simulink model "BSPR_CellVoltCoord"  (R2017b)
settings: Solver=FixedStepDiscrete  StartTime=0.0  StopTime=10.0  FixedStep=0.02  RelTol=1e-3  EnableMultiTasking=on
undefined symbols (not defined in the file): bin2dec, BSPR_CellVoltVldChkDisbl_C, BSPR_cntCellInvldNum_C, BSPR_cntCellSerNum_C, BSPR_cntCellVoltOutRngDiag_CW, BSPR_cntCellVoltVldDiag_CW, BSPR_cntCellVoltVldHi_C, BSPR_cntVoltCellAvl_C, BSPR_iCellVoltDeltaBattCurr_X, BSPR_rCellVoltDeltaBattSOC_Y, BSPR_tBattTempForCellHi_C, BSPR_tBattTempForCellLo_C, BSPR_tiCellVoltInvldChk_C, BSPR_tiCellVoltInvldChkdT_C, BSPR_tiCellVoltRngHiChk_C, BSPR_tiCellVoltRngHiChkdT_C, BSPR_tiCellVoltRngLoChk_C, BSPR_tiCellVoltRngLoChkdT_C, BSPR_uCellVoltDelta_Z, BSPR_uCellVoltHi_C, BSPR_uCellVoltLo_C, BSPR_uCellVoltMaxLim_C, BSPR_uCellVoltMinLim_C
libraries: simulink x35, AIWAYS_Powertrain_BMS_lib x2
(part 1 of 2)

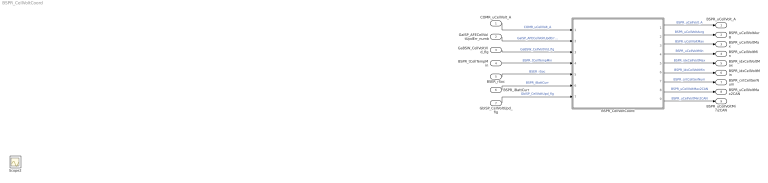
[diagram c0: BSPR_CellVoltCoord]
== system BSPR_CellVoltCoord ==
  COMR_uCellVolt_A : Inport
  GaISP_AFECellVoltUpdErr_numb : Inport  Port=2
  GaBSW_CellVoltVld_flg : Inport  Port=3
  BSPR_tCellTempMin : Inport  Port=4
  BSER_rSoc : Inport  Port=5
  BSPR_iBattCurr : Inport  Port=6
  GbISP_CellVoltUpd_flg : Inport  Port=7
  BSPR_CellVoltCoord : Subsystem
  BSPR_uCellVolt_A : Outport
  BSPR_uCellVoltAvrg : Outport  Port=2
  BSPR_uCellVoltMax : Outport  Port=3
  BSPR_uCellVoltMin : Outport  Port=4
  BSPR_idxCellVoltMax : Outport  Port=5
  BSPR_idxCellVoltMin : Outport  Port=6
  BSPR_cntCellSerNum : Outport  Port=7
  BSPR_uCellVoltMax2CAN : Outport  Port=8
  BSPR_uCellVoltMin2CAN : Outport  Port=9
  Scope2 : Scope
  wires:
  COMR_uCellVolt_A/1 -> BSPR_CellVoltCoord/1(COMR_uCellVolt_A)  "COMR_uCellVolt_A"
  BSPR_CellVoltCoord/1(BSPR_uCellVolt_A) -> BSPR_uCellVolt_A/1  "BSPR_uCellVolt_A"
  BSPR_CellVoltCoord/2(BSPR_uCellVoltAvrg) -> BSPR_uCellVoltAvrg/1  "BSPR_uCellVoltAvrg"
  BSPR_CellVoltCoord/3(BSPR_uCellVoltMax) -> BSPR_uCellVoltMax/1  "BSPR_uCellVoltMax"
  BSPR_CellVoltCoord/4(BSPR_uCellVoltMin) -> BSPR_uCellVoltMin/1  "BSPR_uCellVoltMin"
  BSPR_CellVoltCoord/5(BSPR_idxCellVoltMax) -> BSPR_idxCellVoltMax/1  "BSPR_idxCellVoltMax"
  BSPR_CellVoltCoord/6(BSPR_idxCellVoltMin) -> BSPR_idxCellVoltMin/1  "BSPR_idxCellVoltMin"
  GaISP_AFECellVoltUpdErr_numb/1 -> BSPR_CellVoltCoord/2(GaISP_AFECellVoltUpdErr_numb)  "GaISP_AFECellVoltUpdErr_numb"
  BSPR_CellVoltCoord/7(BSPR_cntCellSerNum) -> BSPR_cntCellSerNum/1  "BSPR_cntCellSerNum"
  GaBSW_CellVoltVld_flg/1 -> BSPR_CellVoltCoord/3(GaBSW_CellVoltVld_flg)  "GaBSW_CellVoltVld_flg"
  BSPR_tCellTempMin/1 -> BSPR_CellVoltCoord/4(BSPR_tCellTempMin)  "BSPR_tCellTempMin"
  BSER_rSoc/1 -> BSPR_CellVoltCoord/5(BSER_rSoc)  "BSER_rSoc"
  BSPR_iBattCurr/1 -> BSPR_CellVoltCoord/6(BSPR_iBattCurr)  "BSPR_iBattCurr"
  BSPR_CellVoltCoord/8(BSPR_uCellVoltMax2CAN) -> BSPR_uCellVoltMax2CAN/1  "BSPR_uCellVoltMax2CAN"
  BSPR_CellVoltCoord/9(BSPR_uCellVoltMin2CAN) -> BSPR_uCellVoltMin2CAN/1  "BSPR_uCellVoltMin2CAN"
  GbISP_CellVoltUpd_flg/1 -> BSPR_CellVoltCoord/7(GbISP_CellVoltUpd_flg)  "GbISP_CellVoltUpd_flg"

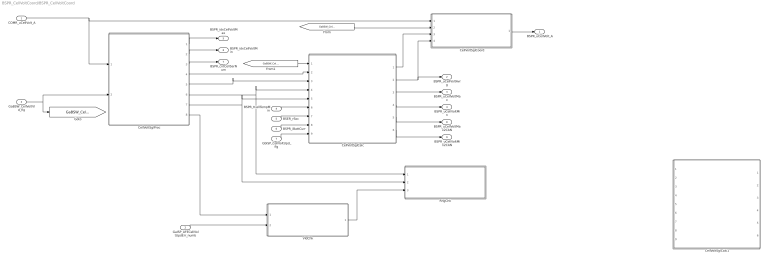
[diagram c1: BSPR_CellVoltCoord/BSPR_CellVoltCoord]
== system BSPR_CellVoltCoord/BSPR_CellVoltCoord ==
  COMR_uCellVolt_A : Inport
  GaISP_AFECellVoltUpdErr_numb : Inport  Port=2
  GaBSW_CellVoltVld_flg : Inport  Port=3
  BSPR_tCellTempMin : Inport  Port=4
  BSER_rSoc : Inport  Port=5
  BSPR_iBattCurr : Inport  Port=6
  GbISP_CellVoltUpd_flg : Inport  Port=7
  CellVoltSglCalc : Subsystem
  CellVoltSglCalc1 : Subsystem  Commented=on
  CellVoltSglCoord : Subsystem
  CellVoltSglProc : Subsystem
  RngChk : Subsystem
  VldChk : Subsystem
  BSPR_uCellVolt_A : Outport
  BSPR_uCellVoltAvrg : Outport  Port=2
  BSPR_uCellVoltMax : Outport  Port=3
  BSPR_uCellVoltMin : Outport  Port=4
  BSPR_idxCellVoltMax : Outport  Port=5
  BSPR_idxCellVoltMin : Outport  Port=6
  BSPR_cntCellSerNum : Outport  Port=7
  BSPR_uCellVoltMax2CAN : Outport  Port=8
  BSPR_uCellVoltMin2CAN : Outport  Port=9
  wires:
  CellVoltSglProc/6(BSPR_uCellVoltMaxTmp) -> RngChk/1(BSPR_uCellVoltMaxTemp), CellVoltSglCalc/4(BSPR_uCellVoltMaxTmp)
  CellVoltSglProc/7(BSPR_uCellVoltMinTmp) -> CellVoltSglCalc/5(BSPR_uCellVoltMinTmp), RngChk/2(BSPR_uCellVoltMinTemp)
  CellVoltSglProc/4(BSPR_uSumVoltCellAvl) -> CellVoltSglCalc/2(BSPR_uSumVoltCellAvl)
  CellVoltSglProc/5(BSPR_cntVoltCellAvl) -> CellVoltSglCalc/3(BSPR_cntVoltCellAvl)
  CellVoltSglProc/1(BSPR_idxCellVoltMax) -> BSPR_idxCellVoltMax/1
  CellVoltSglProc/2(BSPR_idxCellVoltMin) -> BSPR_idxCellVoltMin/1
  CellVoltSglCoord/1(BSPR_uCellVolt_A) -> BSPR_uCellVolt_A/1
  CellVoltSglCalc/2(BSPR_uCellVoltAvrg) -> BSPR_uCellVoltAvrg/1, CellVoltSglCoord/4(BSPR_uCellVoltAvrg)
  CellVoltSglCalc/3(BSPR_uCellVoltMax) -> BSPR_uCellVoltMax/1
  CellVoltSglCalc/4(BSPR_uCellVoltMin) -> BSPR_uCellVoltMin/1
  CellVoltSglProc/8(BSPR_bCellVoltInvld_A) -> VldChk/1(BSPR_bCellVoltInvld_A)
  CellVoltSglProc/3(BSPR_cntCellSerNum) -> BSPR_cntCellSerNum/1
  COMR_uCellVolt_A/1 -> CellVoltSglProc/1(COMR_uCellVolt_A), CellVoltSglCoord/1(COMR_uCellVolt_A)
  VldChk/1(BSPR_bCellVoltElecNorm) -> RngChk/3(BSPR_bCellVoltElecNorm)
  GaBSW_CellVoltVld_flg/1 -> [GaBSW_CellVoltVld_flg], CellVoltSglProc/2(GaBSW_CellVoltVld_flg)
  GaISP_AFECellVoltUpdErr_numb/1 -> VldChk/2(GaISP_AFECellVoltUpdErr_numb)
  [GaBSW_CellVoltVld_flg] -> CellVoltSglCoord/2(GaBSW_CellVoltVld_flg)
  BSPR_tCellTempMin/1 -> CellVoltSglCalc/6(BSPR_tCellTempMin)
  BSER_rSoc/1 -> CellVoltSglCalc/7(BSER_rSoc)
  BSPR_iBattCurr/1 -> CellVoltSglCalc/8(BSPR_iBattCurr)
  CellVoltSglCalc/1(BSPR_bCellVoltInvld_flg) -> CellVoltSglCoord/3(BSPR_bCellVoltInvld_flg)
  [GaBSW_CellVoltVld_flg] -> CellVoltSglCalc/1(GaBSW_CellVoltVld_flg)
  CellVoltSglCalc/5(BSPR_uCellVoltMax2CAN) -> BSPR_uCellVoltMax2CAN/1
  CellVoltSglCalc/6(BSPR_uCellVoltMin2CAN) -> BSPR_uCellVoltMin2CAN/1
  GbISP_CellVoltUpd_flg/1 -> CellVoltSglCalc/9(GbISP_CellVoltUpd_flg)

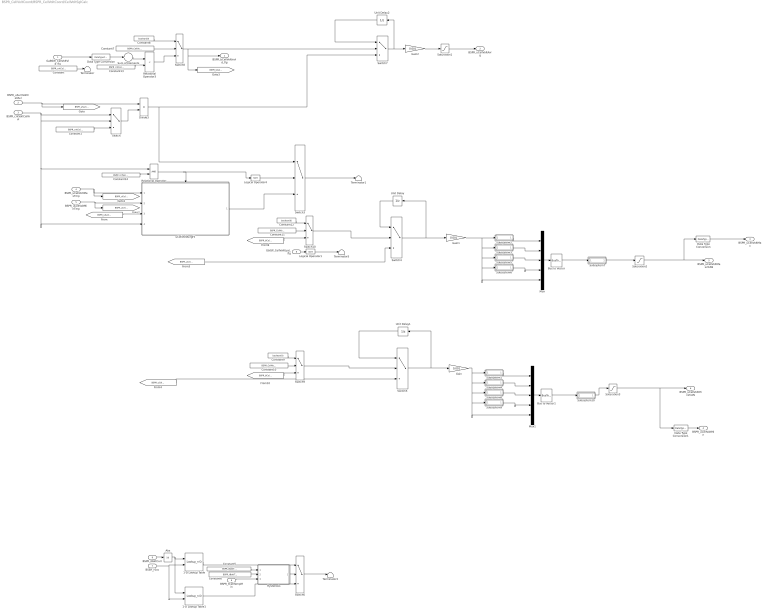
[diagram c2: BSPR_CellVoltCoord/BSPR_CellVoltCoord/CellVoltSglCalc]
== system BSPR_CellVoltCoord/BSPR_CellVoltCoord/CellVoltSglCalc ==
  GaBSW_CellVoltVld_flg : Inport
  BSPR_uSumVoltCellAvl : Inport  Port=2
  BSPR_cntVoltCellAvl : Inport  Port=3
  BSPR_uCellVoltMaxTmp : Inport  Port=4
  BSPR_uCellVoltMinTmp : Inport  Port=5
  BSPR_tCellTempMin : Inport  Port=6
  BSER_rSoc : Inport  Port=7
  BSPR_iBattCurr : Inport  Port=8
  GbISP_CellVoltUpd_flg : Inport  Port=9
  1-D Lookup Table : Lookup_n-D  BreakpointsForDimension1=BSPR_iCellVoltDeltaBattCurr_X  BreakpointsForDimension2=BSPR_rCellVoltDeltaBattSOC_Y  Table=BSPR_uCellVoltDelta_Z  InterpMethod=Flat  ExtrapMethod=Clip  InternalRulePriority=Speed  RndMeth=Simplest
  1-D Lookup Table1 : Lookup_n-D  BreakpointsForDimension1=BSPR_iCellVoltDeltaBattCurr_X  BreakpointsForDimension2=BSPR_rCellVoltDeltaBattSOC_Y  Table=BSPR_uCellVoltDelta_Z  InterpMethod=Flat  ExtrapMethod=Clip  InternalRulePriority=Speed  RndMeth=Simplest
  Abs : Abs
  Bus to Vector : BusToVector
  Bus to Vector1 : BusToVector
  Constant : Constant  Value=BSPR_cntCellSerNum_C
  Constant1 : Constant  Value=BSPR_cntCellSerNum_C
  Constant10 : Constant  Value=BSPR_CellVoltVldChkDisbl_C
  Constant11 : Constant  Value=BSPR_CellVoltVldChkDisbl_C
  Constant12 : Constant  Value=boolean(0)  OutDataTypeStr=boolean
  Constant13 : Constant  Value=BSPR_cntCellInvldNum_C
  Constant14 : Constant  Value=BSPR_cntVoltCellAvl_C
  Constant5 : Constant  Value=BSPR_tBattTempForCellLo_C
  Constant6 : Constant  Value=BSPR_tBattTempForCellHi_C
  Constant7 : Constant  Value=BSPR_CellVoltVldChkDisbl_C
  Constant8 : Constant  Value=boolean(0)  OutDataTypeStr=boolean
  Constant9 : Constant  Value=boolean(0)  OutDataTypeStr=boolean
  Data Type Conversion : DataTypeConversion
  Data Type Conversion1 : DataTypeConversion
  Data Type Conversion : DataTypeConversion  OutDataTypeStr=uint8
  Divide3 : Product  Inputs=*/
  Gain : Gain  Gain=0.001
  Gain1 : Gain  Gain=0.001
  Gain2 : Gain  Gain=0.001
  Hysteresis : Subsystem  TreatAsAtomicUnit=on
  Logical Operator1 : Logic  Operator=NOT  AllPortsSameDT=off  OutDataTypeStr=boolean
  Logical Operator4 : Logic  Operator=NOT  AllPortsSameDT=off  OutDataTypeStr=boolean
  Mux : Mux  Inputs=5
  Mux1 : Mux  Inputs=5
  Relational Operator : RelationalOperator  OutDataTypeStr=boolean  RndMeth=Simplest
  Relational Operator3 : RelationalOperator  Operator=<  OutDataTypeStr=boolean  RndMeth=Simplest
  Saturation1 : Saturate  UpperLimit=BSPR_uCellVoltMaxLim_C  LowerLimit=BSPR_uCellVoltMinLim_C
  Saturation2 : Saturate  UpperLimit=BSPR_uCellVoltMaxLim_C  LowerLimit=BSPR_uCellVoltMinLim_C
  Saturation3 : Saturate  UpperLimit=BSPR_uCellVoltMaxLim_C  LowerLimit=BSPR_uCellVoltMinLim_C
  Subsystem1 : Subsystem
  Subsystem10 : Subsystem  TreatAsAtomicUnit=on  RTWFcnName=RTE_GetMidVal_A  RTWFileName=rte_func
  Subsystem2 : Subsystem
  Subsystem3 : Subsystem
  Subsystem4 : Subsystem
  Subsystem5 : Subsystem
  Subsystem6 : Subsystem
  Subsystem7 : Subsystem  TreatAsAtomicUnit=on  RTWFcnName=RTE_GetMidVal  RTWFileName=rte_func
  Subsystem8 : Subsystem
  Subsystem9 : Subsystem
  Sum of Elements : Sum  Inputs=+
  Switch{,4..10} (8 alike) : Switch  Criteria=u2 ~= 0
  Switch3 : Switch  Criteria=u2 ~= 0  Threshold=2
  Terminator{,1,3,5} (4 alike) : Terminator
  Unit Delay : UnitDelay  SampleTime=-1
  Unit Delay1 : UnitDelay  SampleTime=-1
  Unit Delay2 : UnitDelay  SampleTime=-1
  uCellVoltAvrgFil : Subsystem
  BSPR_bCellVoltInvld_flg : Outport
  BSPR_uCellVoltAvrg : Outport  Port=2
  BSPR_uCellVoltMax : Outport  Port=3
  BSPR_uCellVoltMin : Outport  Port=4
  BSPR_uCellVoltMax2CAN : Outport  Port=5
  BSPR_uCellVoltMin2CAN : Outport  Port=6
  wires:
  Switch7/1 -> Gain2/1, Unit Delay2/1
  BSPR_uSumVoltCellAvl/1 -> [BSPR_uSumVoltCellAvl], Divide3/1
  Saturation1/1 -> BSPR_uCellVoltAvrg/1
  Saturation2/1 -> Data Type Conversion/1, BSPR_uCellVoltMax2CAN/1
  Saturation3/1 -> Data Type Conversion1/1, BSPR_uCellVoltMin2CAN/1
  Constant1/1 -> Switch/3
  Switch/1 -> Divide3/2
  BSPR_cntVoltCellAvl/1 -> uCellVoltAvrgFil/4(BSPR_cntVoltCellAvl), Relational Operator/1, Switch/2, Switch/1
  BSPR_uCellVoltMaxTmp/1 -> [BSPR_uCellVoltMaxTmp], uCellVoltAvrgFil/1(BSPR_uCellVoltMaxTmp)
  BSPR_uCellVoltMinTmp/1 -> [BSPR_uCellVoltMinTmp], uCellVoltAvrgFil/2(BSPR_uCellVoltMinTmp)
  [BSPR_uSumVoltCellAvl] -> uCellVoltAvrgFil/3(BSPR_uSumVoltCellAvl)
  Relational Operator/1 -> uCellVoltAvrgFil/Enable, Logical Operator4/1
  Constant14/1 -> Relational Operator/2
  Logical Operator4/1 -> Switch3/2
  uCellVoltAvrgFil/1(BSPR_uCellVoltAvrgFil) -> Switch3/3
  Switch3/1 -> Terminator1/1
  Unit Delay/1 -> Switch4/1
  Unit Delay1/1 -> Switch5/1
  Switch5/1 -> Unit Delay1/1, Gain/1
  BSPR_tCellTempMin/1 -> Hysteresis/3(u)
  Hysteresis/1(y) -> Switch6/2
  BSPR_iBattCurr/1 -> Abs/1
  BSER_rSoc/1 -> 1-D Lookup Table1/2, 1-D Lookup Table/2
  1-D Lookup Table/1 -> Switch6/1
  Switch6/1 -> Terminator3/1
  1-D Lookup Table1/1 -> Switch6/3
  Abs/1 -> 1-D Lookup Table1/1, 1-D Lookup Table/1
  Constant5/1 -> Hysteresis/1(LSP)
  Constant6/1 -> Hysteresis/2(RSP)
  Data Type Conversion/1 -> Sum of Elements/1
  GaBSW_CellVoltVld_flg/1 -> Data Type Conversion/1
  Sum of Elements/1 -> Relational Operator3/1
  Constant/1 -> Terminator/1
  Switch8/1 -> BSPR_bCellVoltInvld_flg/1, [BSPR_bCellVoltInvld_flg], Switch7/2
  Unit Delay2/1 -> Switch7/1
  Relational Operator3/1 -> Switch8/3
  Constant7/1 -> Switch8/2
  Constant8/1 -> Switch8/1
  Constant10/1 -> Switch9/2
  Constant9/1 -> Switch9/1
  Constant11/1 -> Switch10/2
  Constant12/1 -> Switch10/1
  Constant13/1 -> Relational Operator3/2
  Divide3/1 -> Switch3/1, Switch7/3
  Gain2/1 -> Saturation1/1
  Switch4/1 -> Gain1/1, Unit Delay/1
  Subsystem2/1(y) -> Mux/1
  Subsystem3/1(y) -> Mux/2
  Gain1/1 -> Mux/5, Subsystem6/1(u), Subsystem5/1(u), Subsystem3/1(u), Subsystem2/1(u)
  [BSPR_uCellVoltMaxTmp] -> Switch4/3
  [BSPR_uCellVoltMinTmp] -> Switch5/3
  Data Type Conversion/1 -> BSPR_uCellVoltMax/1
  Data Type Conversion1/1 -> BSPR_uCellVoltMin/1
  [BSPR_bCellVoltInvld_flg] -> Switch10/3
  GbISP_CellVoltUpd_flg/1 -> Logical Operator1/1
  Logical Operator1/1 -> Terminator5/1
  [BSPR_bCellVoltInvld_flg] -> Switch9/3
  Mux/1 -> Bus to Vector/1
  Subsystem5/1(y) -> Mux/3
  Subsystem6/1(y) -> Mux/4
  Bus to Vector/1 -> Subsystem7/1(u)
  Subsystem7/1(y) -> Saturation2/1
  Bus to Vector1/1 -> Subsystem10/1(u)
  Subsystem9/1(y) -> Mux1/4
  Subsystem8/1(y) -> Mux1/3
  Mux1/1 -> Bus to Vector1/1
  Gain/1 -> Subsystem1/1(u), Subsystem4/1(u), Subsystem8/1(u), Subsystem9/1(u), Mux1/5
  Subsystem4/1(y) -> Mux1/2
  Subsystem1/1(y) -> Mux1/1
  Subsystem10/1(y) -> Saturation3/1
  Switch10/1 -> Switch4/2
  Switch9/1 -> Switch5/2

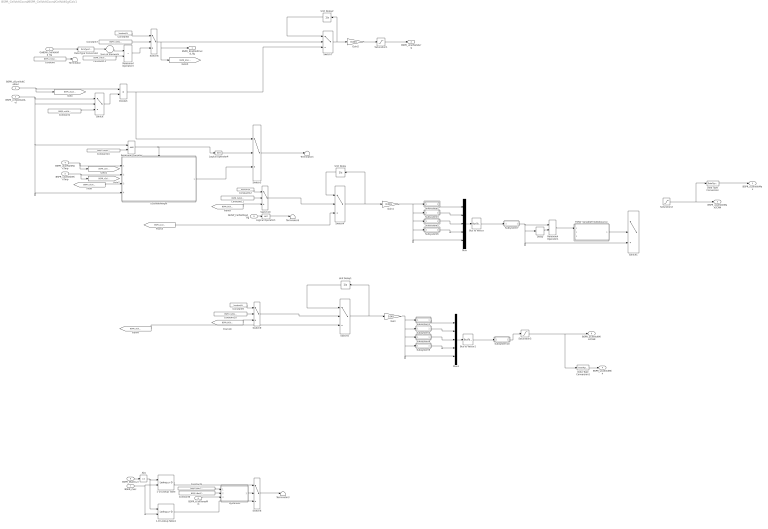
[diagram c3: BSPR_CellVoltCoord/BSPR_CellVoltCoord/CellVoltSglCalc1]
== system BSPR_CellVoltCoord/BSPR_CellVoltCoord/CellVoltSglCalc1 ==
  GaBSW_CellVoltVld_flg : Inport
  BSPR_uSumVoltCellAvl : Inport  Port=2
  BSPR_cntVoltCellAvl : Inport  Port=3
  BSPR_uCellVoltMaxTmp : Inport  Port=4
  BSPR_uCellVoltMinTmp : Inport  Port=5
  BSPR_tCellTempMin : Inport  Port=6
  BSER_rSoc : Inport  Port=7
  BSPR_iBattCurr : Inport  Port=8
  GbISP_CellVoltUpd_flg : Inport  Port=9
  1-D Lookup Table : Lookup_n-D  BreakpointsForDimension1=BSPR_iCellVoltDeltaBattCurr_X  BreakpointsForDimension2=BSPR_rCellVoltDeltaBattSOC_Y  Table=BSPR_uCellVoltDelta_Z  InterpMethod=Flat  ExtrapMethod=Clip  InternalRulePriority=Speed  RndMeth=Simplest
  1-D Lookup Table1 : Lookup_n-D  BreakpointsForDimension1=BSPR_iCellVoltDeltaBattCurr_X  BreakpointsForDimension2=BSPR_rCellVoltDeltaBattSOC_Y  Table=BSPR_uCellVoltDelta_Z  InterpMethod=Flat  ExtrapMethod=Clip  InternalRulePriority=Speed  RndMeth=Simplest
  Abs : Abs
  Bus to Vector : BusToVector
  Bus to Vector1 : BusToVector
  Constant : Constant  Value=BSPR_cntCellSerNum_C
  Constant1 : Constant  Value=BSPR_cntCellSerNum_C
  Constant10 : Constant  Value=BSPR_CellVoltVldChkDisbl_C
  Constant11 : Constant  Value=BSPR_CellVoltVldChkDisbl_C
  Constant12 : Constant  Value=boolean(0)  OutDataTypeStr=boolean
  Constant13 : Constant  Value=BSPR_cntCellInvldNum_C
  Constant14 : Constant  Value=BSPR_cntVoltCellAvl_C
  Constant5 : Constant  Value=BSPR_tBattTempForCellLo_C
  Constant6 : Constant  Value=BSPR_tBattTempForCellHi_C
  Constant7 : Constant  Value=BSPR_CellVoltVldChkDisbl_C
  Constant8 : Constant  Value=boolean(0)  OutDataTypeStr=boolean
  Constant9 : Constant  Value=boolean(0)  OutDataTypeStr=boolean
  Data Type Conversion : DataTypeConversion
  Data Type Conversion1 : DataTypeConversion
  Data Type Conversion : DataTypeConversion  OutDataTypeStr=uint8
  Delay : Delay  DelayLength=1
  Divide3 : Product  Inputs=*/
  Gain : Gain  Gain=0.001
  Gain1 : Gain  Gain=0.001
  Gain2 : Gain  Gain=0.001
  Hysteresis : Subsystem  TreatAsAtomicUnit=on
  Logical Operator1 : Logic  Operator=NOT  AllPortsSameDT=off  OutDataTypeStr=boolean
  Logical Operator4 : Logic  Operator=NOT  AllPortsSameDT=off  OutDataTypeStr=boolean
  Mux : Mux  Inputs=5
  Mux1 : Mux  Inputs=5
  Relational Operator : RelationalOperator  OutDataTypeStr=boolean  RndMeth=Simplest
  Relational Operator1 : RelationalOperator  Operator===  OutDataTypeStr=boolean  RndMeth=Simplest
  Relational Operator3 : RelationalOperator  Operator=<  OutDataTypeStr=boolean  RndMeth=Simplest
  Saturation1 : Saturate  UpperLimit=BSPR_uCellVoltMaxLim_C  LowerLimit=BSPR_uCellVoltMinLim_C
  Saturation2 : Saturate  UpperLimit=BSPR_uCellVoltMaxLim_C  LowerLimit=BSPR_uCellVoltMinLim_C
  Saturation3 : Saturate  UpperLimit=BSPR_uCellVoltMaxLim_C  LowerLimit=BSPR_uCellVoltMinLim_C
  Subsystem1 : Subsystem
  Subsystem10 : Subsystem  TreatAsAtomicUnit=on  RTWFcnName=RTE_GetMidVal_A  RTWFileName=rte_func
  Subsystem2 : Subsystem
  Subsystem3 : Subsystem
  Subsystem4 : Subsystem
  Subsystem5 : Subsystem
  Subsystem6 : Subsystem
  Subsystem7 : Subsystem  TreatAsAtomicUnit=on  RTWFcnName=RTE_GetMidVal  RTWFileName=rte_func
  Subsystem8 : Subsystem
  Subsystem9 : Subsystem
  Sum of Elements : Sum  Inputs=+
  Switch{,4..10} (8 alike) : Switch  Criteria=u2 ~= 0
  Switch1 : Switch  Criteria=u2 ~= 0  Threshold=1  RndMeth=Zero
  Switch3 : Switch  Criteria=u2 ~= 0  Threshold=2
  TONV_VariableTimeDebounce : Subsystem  TreatAsAtomicUnit=on  RTWFcnName=TONV_VariableTimeDebounce  RTWFileName=SrvLib
  Terminator{,1,3,5} (4 alike) : Terminator
  Unit Delay : UnitDelay  SampleTime=-1
  Unit Delay1 : UnitDelay  SampleTime=-1
  Unit Delay2 : UnitDelay  SampleTime=-1
  uCellVoltAvrgFil : Subsystem
  BSPR_bCellVoltInvld_flg : Outport
  BSPR_uCellVoltAvrg : Outport  Port=2
  BSPR_uCellVoltMax : Outport  Port=3
  BSPR_uCellVoltMin : Outport  Port=4
  BSPR_uCellVoltMax2CAN : Outport  Port=5
  BSPR_uCellVoltMin2CAN : Outport  Port=6
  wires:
  Switch7/1 -> Gain2/1, Unit Delay2/1
  BSPR_uSumVoltCellAvl/1 -> [BSPR_uSumVoltCellAvl], Divide3/1
  Saturation1/1 -> BSPR_uCellVoltAvrg/1
  Saturation2/1 -> Data Type Conversion/1, BSPR_uCellVoltMax2CAN/1
  Saturation3/1 -> Data Type Conversion1/1, BSPR_uCellVoltMin2CAN/1
  Constant1/1 -> Switch/3
  Switch/1 -> Divide3/2
  BSPR_cntVoltCellAvl/1 -> uCellVoltAvrgFil/4(BSPR_cntVoltCellAvl), Relational Operator/1, Switch/2, Switch/1
  BSPR_uCellVoltMaxTmp/1 -> [BSPR_uCellVoltMaxTmp], uCellVoltAvrgFil/1(BSPR_uCellVoltMaxTmp)
  BSPR_uCellVoltMinTmp/1 -> [BSPR_uCellVoltMinTmp], uCellVoltAvrgFil/2(BSPR_uCellVoltMinTmp)
  [BSPR_uSumVoltCellAvl] -> uCellVoltAvrgFil/3(BSPR_uSumVoltCellAvl)
  Relational Operator/1 -> uCellVoltAvrgFil/Enable, Logical Operator4/1
  Constant14/1 -> Relational Operator/2
  Logical Operator4/1 -> Switch3/2
  uCellVoltAvrgFil/1(BSPR_uCellVoltAvrgFil) -> Switch3/3
  Switch3/1 -> Terminator1/1
  Unit Delay/1 -> Switch4/1
  Unit Delay1/1 -> Switch5/1
  Switch5/1 -> Unit Delay1/1, Gain/1
  BSPR_tCellTempMin/1 -> Hysteresis/3(u)
  Hysteresis/1(y) -> Switch6/2
  BSPR_iBattCurr/1 -> Abs/1
  BSER_rSoc/1 -> 1-D Lookup Table1/2, 1-D Lookup Table/2
  1-D Lookup Table/1 -> Switch6/1
  Switch6/1 -> Terminator3/1
  1-D Lookup Table1/1 -> Switch6/3
  Abs/1 -> 1-D Lookup Table1/1, 1-D Lookup Table/1
  Constant5/1 -> Hysteresis/1(LSP)
  Constant6/1 -> Hysteresis/2(RSP)
  Data Type Conversion/1 -> Sum of Elements/1
  GaBSW_CellVoltVld_flg/1 -> Data Type Conversion/1
  Sum of Elements/1 -> Relational Operator3/1
  Constant/1 -> Terminator/1
  Switch8/1 -> BSPR_bCellVoltInvld_flg/1, [BSPR_bCellVoltInvld_flg], Switch7/2
  Unit Delay2/1 -> Switch7/1
  Relational Operator3/1 -> Switch8/3
  Constant7/1 -> Switch8/2
  Constant8/1 -> Switch8/1
  Constant10/1 -> Switch9/2
  Constant9/1 -> Switch9/1
  Constant11/1 -> Switch10/2
  Constant12/1 -> Switch10/1
  Constant13/1 -> Relational Operator3/2
  Divide3/1 -> Switch3/1, Switch7/3
  Gain2/1 -> Saturation1/1
  Switch4/1 -> Gain1/1, Unit Delay/1
  Subsystem2/1(y) -> Mux/1
  Subsystem3/1(y) -> Mux/2
  Gain1/1 -> Mux/5, Subsystem6/1(u), Subsystem5/1(u), Subsystem3/1(u), Subsystem2/1(u)
  [BSPR_uCellVoltMaxTmp] -> Switch4/3
  [BSPR_uCellVoltMinTmp] -> Switch5/3
  Data Type Conversion/1 -> BSPR_uCellVoltMax/1
  Data Type Conversion1/1 -> BSPR_uCellVoltMin/1
  [BSPR_bCellVoltInvld_flg] -> Switch10/3
  GbISP_CellVoltUpd_flg/1 -> Logical Operator1/1
  Logical Operator1/1 -> Terminator5/1
  [BSPR_bCellVoltInvld_flg] -> Switch9/3
  Mux/1 -> Bus to Vector/1
  Subsystem5/1(y) -> Mux/3
  Subsystem6/1(y) -> Mux/4
  Bus to Vector/1 -> Subsystem7/1(u)
  Subsystem7/1(y) -> Switch1/3, Delay/1, Relational Operator1/1
  Bus to Vector1/1 -> Subsystem10/1(u)
  Subsystem9/1(y) -> Mux1/4
  Subsystem8/1(y) -> Mux1/3
  Mux1/1 -> Bus to Vector1/1
  Gain/1 -> Subsystem1/1(u), Subsystem4/1(u), Subsystem8/1(u), Subsystem9/1(u), Mux1/5
  Subsystem4/1(y) -> Mux1/2
  Subsystem1/1(y) -> Mux1/1
  Subsystem10/1(y) -> Saturation3/1
  Switch10/1 -> Switch4/2
  Switch9/1 -> Switch5/2
  Delay/1 -> Relational Operator1/2
  Relational Operator1/1 -> TONV_VariableTimeDebounce/1(u)
  TONV_VariableTimeDebounce/1(y) -> Switch1/2

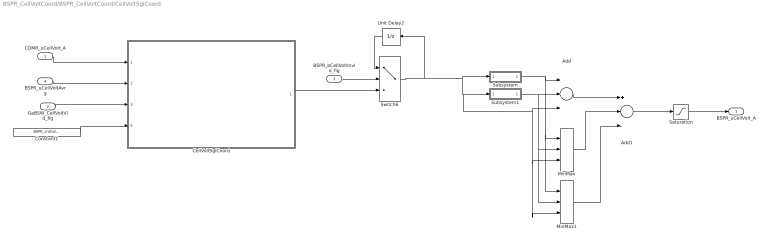
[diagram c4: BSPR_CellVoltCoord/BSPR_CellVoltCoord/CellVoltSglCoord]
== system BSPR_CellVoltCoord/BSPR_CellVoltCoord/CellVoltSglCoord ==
  COMR_uCellVolt_A : Inport
  GaBSW_CellVoltVld_flg : Inport  Port=2
  BSPR_bCellVoltInvld_flg : Inport  Port=3
  BSPR_uCellVoltAvrg : Inport  Port=4
  Add : Sum  Inputs=+++
  Add1 : Sum  Inputs=+--
  CellVoltSglCoord : Stateflow chart  TreatAsAtomicUnit=on
  Constant1 : Constant  Value=BSPR_cntCellSerNum_C
  MinMax : MinMax  Inputs=3
  MinMax1 : MinMax  Function=max  Inputs=3
  Saturation : Saturate  UpperLimit=5  LowerLimit=0
  Subsystem : Subsystem
  Subsystem1 : Subsystem
  Switch6 : Switch  Criteria=u2 ~= 0
  Unit Delay2 : UnitDelay  SampleTime=-1
  BSPR_uCellVolt_A : Outport
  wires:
  COMR_uCellVolt_A/1 -> CellVoltSglCoord/1(COMR_uCellVolt_A)
  BSPR_uCellVoltAvrg/1 -> CellVoltSglCoord/2(BSPR_uCellVoltAvrg)
  Constant1/1 -> CellVoltSglCoord/4(BSPR_cntCellVoltSmpl_C)
  Saturation/1 -> BSPR_uCellVolt_A/1
  GaBSW_CellVoltVld_flg/1 -> CellVoltSglCoord/3(GaBSW_CellVoltVld_flg)
  Subsystem/1(y) -> MinMax1/1, MinMax/1, Add/1
  Subsystem1/1(y) -> Add/2, MinMax/2, MinMax1/2
  Switch6/1 -> Subsystem/1(u), MinMax1/3, MinMax/3, Add/3, Subsystem1/1(u), Unit Delay2/1
  Add/1 -> Add1/1
  MinMax/1 -> Add1/2
  MinMax1/1 -> Add1/3
  Add1/1 -> Saturation/1
  CellVoltSglCoord/1(BSPR_uCellVolt_A) -> Switch6/3
  BSPR_bCellVoltInvld_flg/1 -> Switch6/2
  Unit Delay2/1 -> Switch6/1

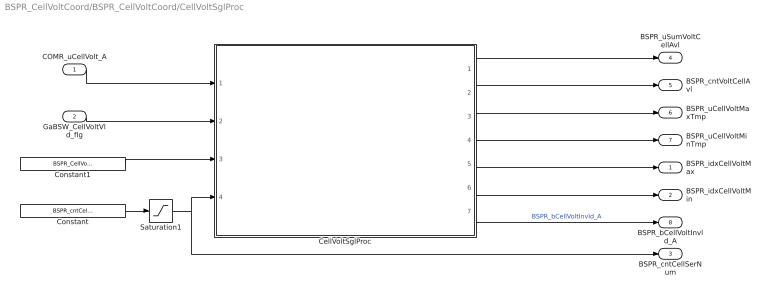
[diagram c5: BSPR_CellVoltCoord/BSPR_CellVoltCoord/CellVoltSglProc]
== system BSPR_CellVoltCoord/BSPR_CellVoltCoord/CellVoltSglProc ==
  COMR_uCellVolt_A : Inport
  GaBSW_CellVoltVld_flg : Inport  Port=2
  CellVoltSglProc : Stateflow chart  TreatAsAtomicUnit=on
  Constant : Constant  Value=BSPR_cntCellSerNum_C
  Constant1 : Constant  Value=BSPR_CellVoltVldChkDisbl_C
  Saturation1 : Saturate  UpperLimit=150  LowerLimit=0
  BSPR_idxCellVoltMax : Outport
  BSPR_idxCellVoltMin : Outport  Port=2
  BSPR_cntCellSerNum : Outport  Port=3
  BSPR_uSumVoltCellAvl : Outport  Port=4
  BSPR_cntVoltCellAvl : Outport  Port=5
  BSPR_uCellVoltMaxTmp : Outport  Port=6
  BSPR_uCellVoltMinTmp : Outport  Port=7
  BSPR_bCellVoltInvld_A : Outport  Port=8
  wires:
  CellVoltSglProc/1(BSPR_uSumVoltCellAvl) -> BSPR_uSumVoltCellAvl/1
  COMR_uCellVolt_A/1 -> CellVoltSglProc/1(COMR_uCellVolt_A)
  CellVoltSglProc/4(BSPR_uCellVoltMinTmp) -> BSPR_uCellVoltMinTmp/1
  CellVoltSglProc/3(BSPR_uCellVoltMaxTmp) -> BSPR_uCellVoltMaxTmp/1
  CellVoltSglProc/2(BSPR_cntVoltCellAvl) -> BSPR_cntVoltCellAvl/1
  CellVoltSglProc/5(BSPR_idxCellVoltMax) -> BSPR_idxCellVoltMax/1
  CellVoltSglProc/6(BSPR_idxCellVoltMin) -> BSPR_idxCellVoltMin/1
  CellVoltSglProc/7(BSPR_bCellVoltInvld_A) -> BSPR_bCellVoltInvld_A/1  "BSPR_bCellVoltInvld_A"
  Constant/1 -> Saturation1/1
  Saturation1/1 -> CellVoltSglProc/4(BSPR_cntCellSerNum_C), BSPR_cntCellSerNum/1
  GaBSW_CellVoltVld_flg/1 -> CellVoltSglProc/2(GaBSW_CellVoltVld_flg)
  Constant1/1 -> CellVoltSglProc/3(BSPR_CellVoltVldChkDisbl_C)

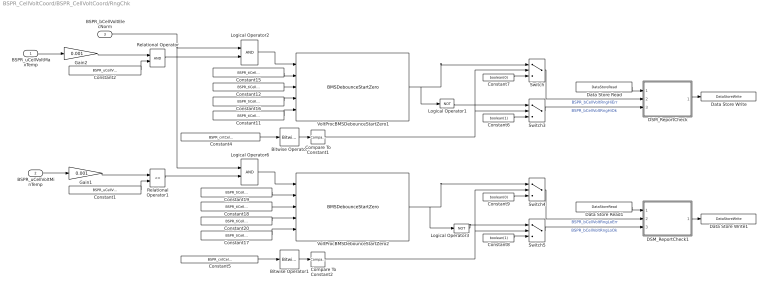
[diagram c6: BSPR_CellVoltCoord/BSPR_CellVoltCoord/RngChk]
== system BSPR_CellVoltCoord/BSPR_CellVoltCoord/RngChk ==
  BSPR_uCellVoltMaxTemp : Inport
  BSPR_uCellVoltMinTemp : Inport  Port=2
  BSPR_bCellVoltElecNorm : Inport  Port=3
  Bitwise Operator : simulink/Logic and Bit Operations/Bitwise Operator  logicop=AND  UseBitMask=on  BitMask=bin2dec('00000001')  BitMaskRealWorld=Stored Integer
  Bitwise Operator1 : simulink/Logic and Bit Operations/Bitwise Operator  logicop=AND  UseBitMask=on  BitMask=bin2dec('00000010')  BitMaskRealWorld=Stored Integer
  Compare To Constant1 : simulink/Logic and Bit Operations/Compare To Constant  relop===  const=1  OutDataTypeStr=boolean
  Compare To Constant2 : simulink/Logic and Bit Operations/Compare To Constant  relop===  const=2  OutDataTypeStr=boolean
  Constant1 : Constant  Value=BSPR_uCellVoltLo_C  OutDataTypeStr=single
  Constant11 : Constant  Value=BSPR_tiCellVoltRngHiChkdT_C  OutDataTypeStr=single
  Constant12 : Constant  Value=BSPR_tiCellVoltRngHiChkdT_C  OutDataTypeStr=single
  Constant15 : Constant  Value=BSPR_tiCellVoltRngHiChk_C  OutDataTypeStr=single
  Constant16 : Constant  Value=BSPR_tiCellVoltRngHiChk_C  OutDataTypeStr=single
  Constant17 : Constant  Value=BSPR_tiCellVoltRngLoChkdT_C  OutDataTypeStr=single
  Constant18 : Constant  Value=BSPR_tiCellVoltRngLoChkdT_C  OutDataTypeStr=single
  Constant19 : Constant  Value=BSPR_tiCellVoltRngLoChk_C  OutDataTypeStr=single
  Constant2 : Constant  Value=BSPR_uCellVoltHi_C  OutDataTypeStr=single
  Constant20 : Constant  Value=BSPR_tiCellVoltRngLoChk_C  OutDataTypeStr=single
  Constant4 : Constant  Value=BSPR_cntCellVoltOutRngDiag_CW
  Constant5 : Constant  Value=BSPR_cntCellVoltOutRngDiag_CW
  Constant6 : Constant  Value=boolean(1)  OutDataTypeStr=boolean
  Constant7 : Constant  Value=boolean(0)  OutDataTypeStr=boolean
  Constant8 : Constant  Value=boolean(1)  OutDataTypeStr=boolean
  Constant9 : Constant  Value=boolean(0)  OutDataTypeStr=boolean
  DSM_ReportCheck : Subsystem  TreatAsAtomicUnit=on  RTWFcnName=DSM_ReportCheck  RTWFileName=SrvLib
  DSM_ReportCheck1 : Subsystem  TreatAsAtomicUnit=on  RTWFcnName=DSM_ReportCheck  RTWFileName=SrvLib
  Data Store Read : DataStoreRead  DataStoreName=DFC_CellVoltRngHiErr
  Data Store Read1 : DataStoreRead  DataStoreName=DFC_CellVoltRngLoErr
  Data Store Write : DataStoreWrite  DataStoreName=DFC_CellVoltRngHiErr
  Data Store Write1 : DataStoreWrite  DataStoreName=DFC_CellVoltRngLoErr
  Gain1 : Gain  Gain=0.001
  Gain2 : Gain  Gain=0.001
  Logical Operator1 : Logic  Operator=NOT  AllPortsSameDT=off  OutDataTypeStr=boolean
  Logical Operator2 : Logic  AllPortsSameDT=off  OutDataTypeStr=boolean
  Logical Operator3 : Logic  Operator=NOT  AllPortsSameDT=off  OutDataTypeStr=boolean
  Logical Operator6 : Logic  AllPortsSameDT=off  OutDataTypeStr=boolean
  Relational Operator : RelationalOperator  OutDataTypeStr=boolean  RndMeth=Simplest
  Relational Operator1 : RelationalOperator  Operator=<=  OutDataTypeStr=boolean  RndMeth=Simplest
  Switch{,3..5} (4 alike) : Switch  Criteria=u2 > Threshold
  VoltProcBMSDebounceStartZero1 : AIWAYS_Powertrain_BMS_lib/Debounce & Delay/BMSDebounceStartZero
  VoltProcBMSDebounceStartZero2 : AIWAYS_Powertrain_BMS_lib/Debounce & Delay/BMSDebounceStartZero
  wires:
  BSPR_uCellVoltMaxTemp/1 -> Gain2/1
  Constant1/1 -> Relational Operator1/2
  Constant2/1 -> Relational Operator/2
  Logical Operator2/1 -> VoltProcBMSDebounceStartZero1/1
  Switch/1 -> DSM_ReportCheck/2(Err)  "BSPR_bCellVoltRngHiErr"
  Switch3/1 -> DSM_ReportCheck/3(Heal)  "BSPR_bCellVoltRngHiOk"
  Data Store Read/1 -> DSM_ReportCheck/1(Dfc_id_nv)
  DSM_ReportCheck/1(Dfc_id) -> Data Store Write/1
  BSPR_uCellVoltMinTemp/1 -> Gain1/1
  Relational Operator/1 -> Logical Operator2/2
  Switch4/1 -> DSM_ReportCheck1/2(Err)  "BSPR_bCellVoltRngLoErr"
  Switch5/1 -> DSM_ReportCheck1/3(Heal)  "BSPR_bCellVoltRngLoOk"
  Data Store Read1/1 -> DSM_ReportCheck1/1(Dfc_id_nv)
  DSM_ReportCheck1/1(Dfc_id) -> Data Store Write1/1
  Relational Operator1/1 -> Logical Operator6/2
  BSPR_bCellVoltElecNorm/1 -> Logical Operator2/1, Logical Operator6/1
  Constant7/1 -> Switch/3
  Constant6/1 -> Switch3/3
  Constant9/1 -> Switch4/3
  Constant8/1 -> Switch5/3
  Bitwise Operator/1 -> Compare To Constant1/1
  Constant4/1 -> Bitwise Operator/1
  Compare To Constant1/1 -> Switch/2, Switch3/2
  Bitwise Operator1/1 -> Compare To Constant2/1
  Constant5/1 -> Bitwise Operator1/1
  Compare To Constant2/1 -> Switch4/2, Switch5/2
  Gain1/1 -> Relational Operator1/1
  Gain2/1 -> Relational Operator/1
  Constant11/1 -> VoltProcBMSDebounceStartZero1/5
  Constant12/1 -> VoltProcBMSDebounceStartZero1/3
  Constant15/1 -> VoltProcBMSDebounceStartZero1/2
  Constant16/1 -> VoltProcBMSDebounceStartZero1/4
  Constant17/1 -> VoltProcBMSDebounceStartZero2/5
  Constant18/1 -> VoltProcBMSDebounceStartZero2/3
  Constant19/1 -> VoltProcBMSDebounceStartZero2/2
  Constant20/1 -> VoltProcBMSDebounceStartZero2/4
  VoltProcBMSDebounceStartZero1/1 -> Logical Operator1/1, Switch/1
  Logical Operator1/1 -> Switch3/1
  Logical Operator6/1 -> VoltProcBMSDebounceStartZero2/1
  VoltProcBMSDebounceStartZero2/1 -> Logical Operator3/1, Switch4/1
  Logical Operator3/1 -> Switch5/1

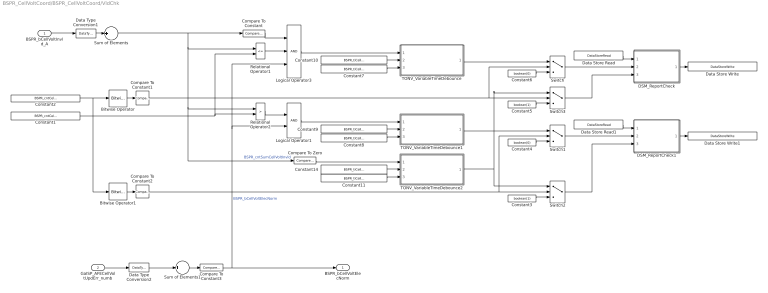
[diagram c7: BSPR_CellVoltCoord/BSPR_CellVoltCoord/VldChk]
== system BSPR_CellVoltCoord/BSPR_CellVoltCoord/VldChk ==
  BSPR_bCellVoltInvld_A : Inport
  GaISP_AFECellVoltUpdErr_numb : Inport  Port=2
  Bitwise Operator : simulink/Logic and Bit Operations/Bitwise Operator  logicop=AND  UseBitMask=on  BitMask=bin2dec('00000001')  BitMaskRealWorld=Stored Integer
  Bitwise Operator1 : simulink/Logic and Bit Operations/Bitwise Operator  logicop=AND  UseBitMask=on  BitMask=bin2dec('00000010')  BitMaskRealWorld=Stored Integer
  Compare To Constant : simulink/Logic and Bit Operations/Compare To Constant  relop=>=  const=1  OutDataTypeStr=boolean
  Compare To Constant1 : simulink/Logic and Bit Operations/Compare To Constant  relop===  const=1  OutDataTypeStr=boolean
  Compare To Constant2 : simulink/Logic and Bit Operations/Compare To Constant  relop===  const=2  OutDataTypeStr=boolean
  Compare To Constant3 : simulink/Logic and Bit Operations/Compare To Constant  relop===  const=0  OutDataTypeStr=boolean
  Compare To Zero : simulink/Logic and Bit Operations/Compare To Zero  relop===  OutDataTypeStr=boolean
  Constant1 : Constant  Value=BSPR_cntCellVoltVldHi_C
  Constant10 : Constant  Value=BSPR_tiCellVoltInvldChk_C  OutDataTypeStr=single
  Constant11 : Constant  Value=BSPR_tiCellVoltInvldChkdT_C  OutDataTypeStr=single
  Constant14 : Constant  Value=BSPR_tiCellVoltInvldChk_C  OutDataTypeStr=single
  Constant2 : Constant  Value=BSPR_cntCellVoltVldDiag_CW
  Constant3 : Constant  Value=boolean(1)  OutDataTypeStr=boolean
  Constant4 : Constant  Value=boolean(0)  OutDataTypeStr=boolean
  Constant5 : Constant  Value=boolean(1)  OutDataTypeStr=boolean
  Constant6 : Constant  Value=boolean(0)  OutDataTypeStr=boolean
  Constant7 : Constant  Value=BSPR_tiCellVoltInvldChkdT_C  OutDataTypeStr=single
  Constant8 : Constant  Value=BSPR_tiCellVoltInvldChkdT_C  OutDataTypeStr=single
  Constant9 : Constant  Value=BSPR_tiCellVoltInvldChk_C  OutDataTypeStr=single
  DSM_ReportCheck : Subsystem  TreatAsAtomicUnit=on  RTWFcnName=DSM_ReportCheck  RTWFileName=SrvLib
  DSM_ReportCheck1 : Subsystem  TreatAsAtomicUnit=on  RTWFcnName=DSM_ReportCheck  RTWFileName=SrvLib
  Data Store Read : DataStoreRead  DataStoreName=DFC_CellVoltVldMin
  Data Store Read1 : DataStoreRead  DataStoreName=DFC_CellVoltVldMax
  Data Store Write : DataStoreWrite  DataStoreName=DFC_CellVoltVldMin
  Data Store Write1 : DataStoreWrite  DataStoreName=DFC_CellVoltVldMax
  Data Type Conversion1 : DataTypeConversion  OutDataTypeStr=uint8
  Data Type Conversion2 : DataTypeConversion  OutDataTypeStr=uint8
  Logical Operator1 : Logic  AllPortsSameDT=off  OutDataTypeStr=boolean
  Logical Operator3 : Logic  Inputs=3  AllPortsSameDT=off  OutDataTypeStr=boolean
  Relational Operator1 : RelationalOperator  Operator=<=  OutDataTypeStr=boolean  RndMeth=Simplest
  Relational Operator2 : RelationalOperator  Operator=>  OutDataTypeStr=boolean  RndMeth=Simplest
  Sum of Elements : Sum  Inputs=+
  Sum of Elements1 : Sum  Inputs=+  OutDataTypeStr=uint8
  Switch{,1..3} (4 alike) : Switch  Criteria=u2 > Threshold
  TONV_VariableTimeDebounce : Subsystem  TreatAsAtomicUnit=on  RTWFcnName=TONV_VariableTimeDebounce  RTWFileName=SrvLib
  TONV_VariableTimeDebounce1 : Subsystem  TreatAsAtomicUnit=on  RTWFcnName=TONV_VariableTimeDebounce  RTWFileName=SrvLib
  TONV_VariableTimeDebounce2 : Subsystem  TreatAsAtomicUnit=on  RTWFcnName=TONV_VariableTimeDebounce  RTWFileName=SrvLib
  BSPR_bCellVoltElecNorm : Outport
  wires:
  Data Store Read/1 -> DSM_ReportCheck/1(Dfc_id_nv)
  DSM_ReportCheck/1(Dfc_id) -> Data Store Write/1
  BSPR_bCellVoltInvld_A/1 -> Data Type Conversion1/1
  Compare To Constant/1 -> Logical Operator3/1
  Constant1/1 -> Relational Operator2/2, Relational Operator1/2
  Relational Operator1/1 -> Logical Operator3/2
  Data Store Read1/1 -> DSM_ReportCheck1/1(Dfc_id_nv)
  DSM_ReportCheck1/1(Dfc_id) -> Data Store Write1/1
  Sum of Elements/1 -> Relational Operator1/1, Relational Operator2/1, Compare To Zero/1, Compare To Constant/1  "BSPR_cntSumCellVoltInvld"
  TONV_VariableTimeDebounce2/1(y) -> Switch3/1, Switch2/1
  Switch/1 -> DSM_ReportCheck/2(Err)
  Switch1/1 -> DSM_ReportCheck1/2(Err)
  Switch2/1 -> DSM_ReportCheck1/3(Heal)
  Switch3/1 -> DSM_ReportCheck/3(Heal)
  Bitwise Operator/1 -> Compare To Constant1/1
  Bitwise Operator1/1 -> Compare To Constant2/1
  Constant2/1 -> Bitwise Operator1/1, Bitwise Operator/1
  Compare To Constant1/1 -> Switch/2, Switch3/2
  Compare To Constant2/1 -> Switch1/2, Switch2/2
  Constant4/1 -> Switch1/3
  Constant3/1 -> Switch2/3
  Constant6/1 -> Switch/3
  Constant5/1 -> Switch3/3
  Relational Operator2/1 -> Logical Operator1/1
  Sum of Elements1/1 -> Compare To Constant3/1
  Compare To Constant3/1 -> Logical Operator3/3, Logical Operator1/2, BSPR_bCellVoltElecNorm/1  "BSPR_bCellVoltElecNorm"
  GaISP_AFECellVoltUpdErr_numb/1 -> Data Type Conversion2/1
  Data Type Conversion1/1 -> Sum of Elements/1
  Data Type Conversion2/1 -> Sum of Elements1/1
  Constant7/1 -> TONV_VariableTimeDebounce/3(dT)
  Constant10/1 -> TONV_VariableTimeDebounce/2(T)
  Logical Operator3/1 -> TONV_VariableTimeDebounce/1(u)
  TONV_VariableTimeDebounce/1(y) -> Switch/1
  Constant8/1 -> TONV_VariableTimeDebounce1/3(dT)
  Constant9/1 -> TONV_VariableTimeDebounce1/2(T)
  Logical Operator1/1 -> TONV_VariableTimeDebounce1/1(u)
  TONV_VariableTimeDebounce1/1(y) -> Switch1/1
  Constant11/1 -> TONV_VariableTimeDebounce2/3(dT)
  Compare To Zero/1 -> TONV_VariableTimeDebounce2/1(u)
  Constant14/1 -> TONV_VariableTimeDebounce2/2(T)

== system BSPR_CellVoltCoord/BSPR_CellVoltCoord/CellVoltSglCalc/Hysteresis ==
  note: Hysteresis
  LSP : Inport
  RSP : Inport  Port=2
  u : Inport  Port=3
  Constant Value : Constant  OutDataTypeStr=boolean
  Constant Value1 : Constant  Value=0  OutDataTypeStr=boolean
  Greater Than : RelationalOperator  Operator=>  OutDataTypeStr=boolean
  Greater Than1 : RelationalOperator  Operator=<  OutDataTypeStr=boolean
  Switch1 : Switch  Criteria=u2 ~= 0  Threshold=1  RndMeth=Zero
  Switch2 : Switch  Criteria=u2 ~= 0  Threshold=1  RndMeth=Zero
  Unit Delay : UnitDelay  SampleTime=-1
  y : Outport
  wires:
  RSP/1 -> Greater Than/2
  LSP/1 -> Greater Than1/2
  Greater Than1/1 -> Switch2/2
  Greater Than/1 -> Switch1/2
  u/1 -> Greater Than1/1, Greater Than/1
  Constant Value/1 -> Switch1/1
  Switch2/1 -> Switch1/3
  Constant Value1/1 -> Switch2/1
  Switch1/1 -> y/1, Unit Delay/1
  Unit Delay/1 -> Switch2/3

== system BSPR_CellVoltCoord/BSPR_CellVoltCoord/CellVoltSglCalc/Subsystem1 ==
  u : Inport
  Constant : Constant  Value=0  OutDataTypeStr=boolean
  Switch : Switch  Criteria=u2 ~= 0
  Unit Delay : UnitDelay  InitialCondition=1  SampleTime=-1
  Unit Delay1 : UnitDelay  SampleTime=-1
  y : Outport
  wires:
  Unit Delay1/1 -> Switch/3
  u/1 -> Switch/1, Unit Delay1/1
  Constant/1 -> Unit Delay/1
  Switch/1 -> y/1
  Unit Delay/1 -> Switch/2

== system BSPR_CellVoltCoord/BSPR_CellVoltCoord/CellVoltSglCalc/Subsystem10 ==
  u : Inport  OutDataTypeStr=single  PortDimensions=5
  Min : MinMax
  y : Outport  OutDataTypeStr=single
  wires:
  u/1 -> Min/1
  Min/1 -> y/1

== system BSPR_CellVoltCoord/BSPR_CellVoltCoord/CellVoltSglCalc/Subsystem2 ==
  u : Inport
  Constant : Constant  Value=0  OutDataTypeStr=boolean
  Switch : Switch  Criteria=u2 ~= 0
  Unit Delay : UnitDelay  InitialCondition=1  SampleTime=-1
  Unit Delay1 : UnitDelay  SampleTime=-1
  y : Outport
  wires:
  Unit Delay/1 -> Switch/2
  Switch/1 -> y/1
  Constant/1 -> Unit Delay/1
  u/1 -> Unit Delay1/1, Switch/1
  Unit Delay1/1 -> Switch/3

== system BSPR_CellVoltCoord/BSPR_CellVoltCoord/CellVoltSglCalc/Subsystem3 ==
  u : Inport
  Constant : Constant  Value=0  OutDataTypeStr=boolean
  Switch : Switch  Criteria=u2 ~= 0
  Unit Delay : UnitDelay  InitialCondition=1  SampleTime=-1
  Unit Delay1 : UnitDelay  SampleTime=-1
  Unit Delay2 : UnitDelay  InitialCondition=1  SampleTime=-1
  Unit Delay3 : UnitDelay  SampleTime=-1
  y : Outport
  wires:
  Unit Delay1/1 -> Unit Delay3/1
  u/1 -> Switch/1, Unit Delay1/1
  Constant/1 -> Unit Delay/1
  Switch/1 -> y/1
  Unit Delay/1 -> Unit Delay2/1
  Unit Delay2/1 -> Switch/2
  Unit Delay3/1 -> Switch/3

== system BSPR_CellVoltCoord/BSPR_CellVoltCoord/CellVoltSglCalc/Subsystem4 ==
  u : Inport
  Constant : Constant  Value=0  OutDataTypeStr=boolean
  Switch : Switch  Criteria=u2 ~= 0
  Unit Delay : UnitDelay  InitialCondition=1  SampleTime=-1
  Unit Delay1 : UnitDelay  SampleTime=-1
  Unit Delay2 : UnitDelay  InitialCondition=1  SampleTime=-1
  Unit Delay3 : UnitDelay  SampleTime=-1
  y : Outport
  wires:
  Unit Delay3/1 -> Switch/3
  Unit Delay2/1 -> Switch/2
  Unit Delay/1 -> Unit Delay2/1
  Switch/1 -> y/1
  Constant/1 -> Unit Delay/1
  u/1 -> Unit Delay1/1, Switch/1
  Unit Delay1/1 -> Unit Delay3/1

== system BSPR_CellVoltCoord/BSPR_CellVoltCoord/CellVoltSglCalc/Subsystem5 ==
  u : Inport
  Constant : Constant  Value=0  OutDataTypeStr=boolean
  Switch : Switch  Criteria=u2 ~= 0
  Unit Delay : UnitDelay  InitialCondition=1  SampleTime=-1
  Unit Delay{1,3..5} (4 alike) : UnitDelay  SampleTime=-1
  Unit Delay2 : UnitDelay  InitialCondition=1  SampleTime=-1
  y : Outport
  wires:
  Unit Delay1/1 -> Unit Delay3/1
  u/1 -> Switch/1, Unit Delay1/1
  Constant/1 -> Unit Delay/1
  Switch/1 -> y/1
  Unit Delay/1 -> Unit Delay2/1
  Unit Delay2/1 -> Unit Delay5/1
  Unit Delay3/1 -> Unit Delay4/1
  Unit Delay4/1 -> Switch/3
  Unit Delay5/1 -> Switch/2

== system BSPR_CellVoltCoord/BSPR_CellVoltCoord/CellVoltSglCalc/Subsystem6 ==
  u : Inport
  Constant : Constant  Value=0  OutDataTypeStr=boolean
  Switch : Switch  Criteria=u2 ~= 0
  Unit Delay : UnitDelay  InitialCondition=1  SampleTime=-1
  Unit Delay{1,3..7} (6 alike) : UnitDelay  SampleTime=-1
  Unit Delay2 : UnitDelay  InitialCondition=1  SampleTime=-1
  y : Outport
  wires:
  Unit Delay1/1 -> Unit Delay3/1
  u/1 -> Switch/1, Unit Delay1/1
  Constant/1 -> Unit Delay/1
  Switch/1 -> y/1
  Unit Delay/1 -> Unit Delay2/1
  Unit Delay2/1 -> Unit Delay5/1
  Unit Delay3/1 -> Unit Delay4/1
  Unit Delay4/1 -> Unit Delay6/1
  Unit Delay5/1 -> Unit Delay7/1
  Unit Delay6/1 -> Switch/3
  Unit Delay7/1 -> Switch/2

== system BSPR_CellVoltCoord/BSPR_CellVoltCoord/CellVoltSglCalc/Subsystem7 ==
  u : Inport  OutDataTypeStr=single  PortDimensions=5
  Min : MinMax
  y : Outport  OutDataTypeStr=single
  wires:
  u/1 -> Min/1
  Min/1 -> y/1

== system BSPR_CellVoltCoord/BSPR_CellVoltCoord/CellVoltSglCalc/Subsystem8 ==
  u : Inport
  Constant : Constant  Value=0  OutDataTypeStr=boolean
  Switch : Switch  Criteria=u2 ~= 0
  Unit Delay : UnitDelay  InitialCondition=1  SampleTime=-1
  Unit Delay{1,3..5} (4 alike) : UnitDelay  SampleTime=-1
  Unit Delay2 : UnitDelay  InitialCondition=1  SampleTime=-1
  y : Outport
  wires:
  Unit Delay5/1 -> Switch/2
  Unit Delay4/1 -> Switch/3
  Unit Delay3/1 -> Unit Delay4/1
  Unit Delay2/1 -> Unit Delay5/1
  Unit Delay/1 -> Unit Delay2/1
  Switch/1 -> y/1
  Constant/1 -> Unit Delay/1
  u/1 -> Unit Delay1/1, Switch/1
  Unit Delay1/1 -> Unit Delay3/1

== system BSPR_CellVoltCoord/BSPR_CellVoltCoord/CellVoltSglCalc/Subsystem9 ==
  u : Inport
  Constant : Constant  Value=0  OutDataTypeStr=boolean
  Switch : Switch  Criteria=u2 ~= 0
  Unit Delay : UnitDelay  InitialCondition=1  SampleTime=-1
  Unit Delay{1,3..7} (6 alike) : UnitDelay  SampleTime=-1
  Unit Delay2 : UnitDelay  InitialCondition=1  SampleTime=-1
  y : Outport
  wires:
  Unit Delay7/1 -> Switch/2
  Unit Delay6/1 -> Switch/3
  Unit Delay5/1 -> Unit Delay7/1
  Unit Delay4/1 -> Unit Delay6/1
  Unit Delay3/1 -> Unit Delay4/1
  Unit Delay2/1 -> Unit Delay5/1
  Unit Delay/1 -> Unit Delay2/1
  Switch/1 -> y/1
  Constant/1 -> Unit Delay/1
  u/1 -> Unit Delay1/1, Switch/1
  Unit Delay1/1 -> Unit Delay3/1

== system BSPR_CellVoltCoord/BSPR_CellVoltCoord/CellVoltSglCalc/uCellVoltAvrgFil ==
  BSPR_uCellVoltMaxTmp : Inport
  BSPR_uCellVoltMinTmp : Inport  Port=2
  BSPR_uSumVoltCellAvl : Inport  Port=3
  BSPR_cntVoltCellAvl : Inport  Port=4
  Enable : EnablePort  StatesWhenEnabling=reset
  Add : Sum  Inputs=+-
  Add1 : Sum  Inputs=+--
  Constant5 : Constant  Value=2  OutDataTypeStr=uint8
  Divide1 : Product  Inputs=*/
  BSPR_uCellVoltAvrgFil : Outport
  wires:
  Add1/1 -> Divide1/1
  Constant5/1 -> Add/2
  BSPR_uCellVoltMinTmp/1 -> Add1/3
  BSPR_uCellVoltMaxTmp/1 -> Add1/2
  Divide1/1 -> BSPR_uCellVoltAvrgFil/1  "BSPR_uCellVoltAvrgFil"
  BSPR_cntVoltCellAvl/1 -> Add/1
  Add/1 -> Divide1/2
  BSPR_uSumVoltCellAvl/1 -> Add1/1

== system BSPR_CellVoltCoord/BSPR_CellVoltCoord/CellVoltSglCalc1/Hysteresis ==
  note: Hysteresis
  LSP : Inport
  RSP : Inport  Port=2
  u : Inport  Port=3
  Constant Value : Constant  OutDataTypeStr=boolean
  Constant Value1 : Constant  Value=0  OutDataTypeStr=boolean
  Greater Than : RelationalOperator  Operator=>  OutDataTypeStr=boolean
  Greater Than1 : RelationalOperator  Operator=<  OutDataTypeStr=boolean
  Switch1 : Switch  Criteria=u2 ~= 0  Threshold=1  RndMeth=Zero
  Switch2 : Switch  Criteria=u2 ~= 0  Threshold=1  RndMeth=Zero
  Unit Delay : UnitDelay  SampleTime=-1
  y : Outport
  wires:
  RSP/1 -> Greater Than/2
  LSP/1 -> Greater Than1/2
  Greater Than1/1 -> Switch2/2
  Greater Than/1 -> Switch1/2
  u/1 -> Greater Than1/1, Greater Than/1
  Constant Value/1 -> Switch1/1
  Switch2/1 -> Switch1/3
  Constant Value1/1 -> Switch2/1
  Switch1/1 -> y/1, Unit Delay/1
  Unit Delay/1 -> Switch2/3

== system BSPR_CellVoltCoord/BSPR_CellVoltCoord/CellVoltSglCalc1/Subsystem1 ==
  u : Inport
  Constant : Constant  Value=0  OutDataTypeStr=boolean
  Switch : Switch  Criteria=u2 ~= 0
  Unit Delay : UnitDelay  InitialCondition=1  SampleTime=-1
  Unit Delay1 : UnitDelay  SampleTime=-1
  y : Outport
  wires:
  Unit Delay1/1 -> Switch/3
  u/1 -> Switch/1, Unit Delay1/1
  Constant/1 -> Unit Delay/1
  Switch/1 -> y/1
  Unit Delay/1 -> Switch/2

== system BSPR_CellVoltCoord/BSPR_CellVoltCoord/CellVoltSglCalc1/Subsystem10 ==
  u : Inport  OutDataTypeStr=single  PortDimensions=5
  Min : MinMax
  y : Outport  OutDataTypeStr=single
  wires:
  u/1 -> Min/1
  Min/1 -> y/1

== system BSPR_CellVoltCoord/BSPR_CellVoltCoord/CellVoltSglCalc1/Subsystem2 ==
  u : Inport
  Constant : Constant  Value=0  OutDataTypeStr=boolean
  Switch : Switch  Criteria=u2 ~= 0
  Unit Delay : UnitDelay  InitialCondition=1  SampleTime=-1
  Unit Delay1 : UnitDelay  SampleTime=-1
  y : Outport
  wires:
  Unit Delay/1 -> Switch/2
  Switch/1 -> y/1
  Constant/1 -> Unit Delay/1
  u/1 -> Unit Delay1/1, Switch/1
  Unit Delay1/1 -> Switch/3

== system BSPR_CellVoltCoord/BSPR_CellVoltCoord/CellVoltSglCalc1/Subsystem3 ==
  u : Inport
  Constant : Constant  Value=0  OutDataTypeStr=boolean
  Switch : Switch  Criteria=u2 ~= 0
  Unit Delay : UnitDelay  InitialCondition=1  SampleTime=-1
  Unit Delay1 : UnitDelay  SampleTime=-1
  Unit Delay2 : UnitDelay  InitialCondition=1  SampleTime=-1
  Unit Delay3 : UnitDelay  SampleTime=-1
  y : Outport
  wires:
  Unit Delay1/1 -> Unit Delay3/1
  u/1 -> Switch/1, Unit Delay1/1
  Constant/1 -> Unit Delay/1
  Switch/1 -> y/1
  Unit Delay/1 -> Unit Delay2/1
  Unit Delay2/1 -> Switch/2
  Unit Delay3/1 -> Switch/3

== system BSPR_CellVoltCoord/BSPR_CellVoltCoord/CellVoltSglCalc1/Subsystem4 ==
  u : Inport
  Constant : Constant  Value=0  OutDataTypeStr=boolean
  Switch : Switch  Criteria=u2 ~= 0
  Unit Delay : UnitDelay  InitialCondition=1  SampleTime=-1
  Unit Delay1 : UnitDelay  SampleTime=-1
  Unit Delay2 : UnitDelay  InitialCondition=1  SampleTime=-1
  Unit Delay3 : UnitDelay  SampleTime=-1
  y : Outport
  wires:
  Unit Delay3/1 -> Switch/3
  Unit Delay2/1 -> Switch/2
  Unit Delay/1 -> Unit Delay2/1
  Switch/1 -> y/1
  Constant/1 -> Unit Delay/1
  u/1 -> Unit Delay1/1, Switch/1
  Unit Delay1/1 -> Unit Delay3/1

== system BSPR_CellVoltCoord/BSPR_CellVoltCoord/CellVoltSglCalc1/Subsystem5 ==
  u : Inport
  Constant : Constant  Value=0  OutDataTypeStr=boolean
  Switch : Switch  Criteria=u2 ~= 0
  Unit Delay : UnitDelay  InitialCondition=1  SampleTime=-1
  Unit Delay{1,3..5} (4 alike) : UnitDelay  SampleTime=-1
  Unit Delay2 : UnitDelay  InitialCondition=1  SampleTime=-1
  y : Outport
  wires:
  Unit Delay1/1 -> Unit Delay3/1
  u/1 -> Switch/1, Unit Delay1/1
  Constant/1 -> Unit Delay/1
  Switch/1 -> y/1
  Unit Delay/1 -> Unit Delay2/1
  Unit Delay2/1 -> Unit Delay5/1
  Unit Delay3/1 -> Unit Delay4/1
  Unit Delay4/1 -> Switch/3
  Unit Delay5/1 -> Switch/2

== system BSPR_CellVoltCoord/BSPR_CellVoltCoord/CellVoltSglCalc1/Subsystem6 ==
  u : Inport
  Constant : Constant  Value=0  OutDataTypeStr=boolean
  Switch : Switch  Criteria=u2 ~= 0
  Unit Delay : UnitDelay  InitialCondition=1  SampleTime=-1
  Unit Delay{1,3..7} (6 alike) : UnitDelay  SampleTime=-1
  Unit Delay2 : UnitDelay  InitialCondition=1  SampleTime=-1
  y : Outport
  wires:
  Unit Delay1/1 -> Unit Delay3/1
  u/1 -> Switch/1, Unit Delay1/1
  Constant/1 -> Unit Delay/1
  Switch/1 -> y/1
  Unit Delay/1 -> Unit Delay2/1
  Unit Delay2/1 -> Unit Delay5/1
  Unit Delay3/1 -> Unit Delay4/1
  Unit Delay4/1 -> Unit Delay6/1
  Unit Delay5/1 -> Unit Delay7/1
  Unit Delay6/1 -> Switch/3
  Unit Delay7/1 -> Switch/2

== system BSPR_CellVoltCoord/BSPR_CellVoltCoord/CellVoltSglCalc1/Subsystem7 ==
  u : Inport  OutDataTypeStr=single  PortDimensions=5
  Min : MinMax
  y : Outport  OutDataTypeStr=single
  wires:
  u/1 -> Min/1
  Min/1 -> y/1

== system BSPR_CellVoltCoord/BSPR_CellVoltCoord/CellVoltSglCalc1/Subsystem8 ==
  u : Inport
  Constant : Constant  Value=0  OutDataTypeStr=boolean
  Switch : Switch  Criteria=u2 ~= 0
  Unit Delay : UnitDelay  InitialCondition=1  SampleTime=-1
  Unit Delay{1,3..5} (4 alike) : UnitDelay  SampleTime=-1
  Unit Delay2 : UnitDelay  InitialCondition=1  SampleTime=-1
  y : Outport
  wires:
  Unit Delay5/1 -> Switch/2
  Unit Delay4/1 -> Switch/3
  Unit Delay3/1 -> Unit Delay4/1
  Unit Delay2/1 -> Unit Delay5/1
  Unit Delay/1 -> Unit Delay2/1
  Switch/1 -> y/1
  Constant/1 -> Unit Delay/1
  u/1 -> Unit Delay1/1, Switch/1
  Unit Delay1/1 -> Unit Delay3/1

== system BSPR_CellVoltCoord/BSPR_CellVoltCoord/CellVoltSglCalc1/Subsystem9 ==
  u : Inport
  Constant : Constant  Value=0  OutDataTypeStr=boolean
  Switch : Switch  Criteria=u2 ~= 0
  Unit Delay : UnitDelay  InitialCondition=1  SampleTime=-1
  Unit Delay{1,3..7} (6 alike) : UnitDelay  SampleTime=-1
  Unit Delay2 : UnitDelay  InitialCondition=1  SampleTime=-1
  y : Outport
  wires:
  Unit Delay7/1 -> Switch/2
  Unit Delay6/1 -> Switch/3
  Unit Delay5/1 -> Unit Delay7/1
  Unit Delay4/1 -> Unit Delay6/1
  Unit Delay3/1 -> Unit Delay4/1
  Unit Delay2/1 -> Unit Delay5/1
  Unit Delay/1 -> Unit Delay2/1
  Switch/1 -> y/1
  Constant/1 -> Unit Delay/1
  u/1 -> Unit Delay1/1, Switch/1
  Unit Delay1/1 -> Unit Delay3/1

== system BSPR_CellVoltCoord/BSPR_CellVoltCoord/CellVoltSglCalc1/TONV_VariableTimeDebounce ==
  note: Turn On Delay Time Deboune
  u : Inport
  T : Inport  Port=2
  dT : Inport  Port=3
  Add : Sum
  Constant1 : Constant  Value=0  OutDataTypeStr=single
  Constant2 : Constant  OutDataTypeStr=uint8
  Constant3 : Constant  Value=0  OutDataTypeStr=uint8
  Delay : Delay  DelayLength=1  InitialCondition=0
  MinMax : MinMax  Inputs=2
  Product : Product  OutMin=[0]  OutMax=[65535]  OutDataTypeStr=single
  Relational Operator : RelationalOperator  Operator=>  OutDataTypeStr=boolean  RndMeth=Simplest
  Switch : Switch  Criteria=u2 ~= 0
  Switch1 : Switch  Criteria=u2 ~= 0
  y : Outport
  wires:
  Switch1/1 -> Product/1
  Constant3/1 -> Switch1/3
  Constant2/1 -> Switch1/1
  u/1 -> Switch1/2, Switch/2
  dT/1 -> Switch/1
  Constant1/1 -> Switch/3
  Add/1 -> Product/2
  Product/1 -> Relational Operator/1, Delay/1
  Switch/1 -> Add/1
  Delay/1 -> MinMax/2
  Relational Operator/1 -> y/1
  T/1 -> MinMax/1, Relational Operator/2
  MinMax/1 -> Add/2

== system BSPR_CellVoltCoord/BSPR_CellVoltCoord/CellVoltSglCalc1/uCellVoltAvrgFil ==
  BSPR_uCellVoltMaxTmp : Inport
  BSPR_uCellVoltMinTmp : Inport  Port=2
  BSPR_uSumVoltCellAvl : Inport  Port=3
  BSPR_cntVoltCellAvl : Inport  Port=4
  Enable : EnablePort  StatesWhenEnabling=reset
  Add : Sum  Inputs=+-
  Add1 : Sum  Inputs=+--
  Constant5 : Constant  Value=2  OutDataTypeStr=uint8
  Divide1 : Product  Inputs=*/
  BSPR_uCellVoltAvrgFil : Outport
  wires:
  Add1/1 -> Divide1/1
  Constant5/1 -> Add/2
  BSPR_uCellVoltMinTmp/1 -> Add1/3
  BSPR_uCellVoltMaxTmp/1 -> Add1/2
  Divide1/1 -> BSPR_uCellVoltAvrgFil/1  "BSPR_uCellVoltAvrgFil"
  BSPR_cntVoltCellAvl/1 -> Add/1
  Add/1 -> Divide1/2
  BSPR_uSumVoltCellAvl/1 -> Add1/1

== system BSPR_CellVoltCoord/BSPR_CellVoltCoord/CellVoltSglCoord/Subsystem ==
  u : Inport
  Constant : Constant  Value=0  OutDataTypeStr=boolean
  Switch : Switch  Criteria=u2 ~= 0
  Unit Delay : UnitDelay  InitialCondition=1  SampleTime=-1
  Unit Delay1 : UnitDelay  SampleTime=-1
  y : Outport
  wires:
  Unit Delay/1 -> Switch/2
  Switch/1 -> y/1
  Constant/1 -> Unit Delay/1
  u/1 -> Unit Delay1/1, Switch/1
  Unit Delay1/1 -> Switch/3

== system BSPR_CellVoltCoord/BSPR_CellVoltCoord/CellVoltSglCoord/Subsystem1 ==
  u : Inport
  Constant : Constant  Value=0  OutDataTypeStr=boolean
  Switch : Switch  Criteria=u2 ~= 0
  Unit Delay : UnitDelay  InitialCondition=1  SampleTime=-1
  Unit Delay1 : UnitDelay  SampleTime=-1
  Unit Delay2 : UnitDelay  InitialCondition=1  SampleTime=-1
  Unit Delay3 : UnitDelay  SampleTime=-1
  y : Outport
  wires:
  Unit Delay1/1 -> Unit Delay3/1
  u/1 -> Switch/1, Unit Delay1/1
  Constant/1 -> Unit Delay/1
  Switch/1 -> y/1
  Unit Delay/1 -> Unit Delay2/1
  Unit Delay2/1 -> Switch/2
  Unit Delay3/1 -> Switch/3
